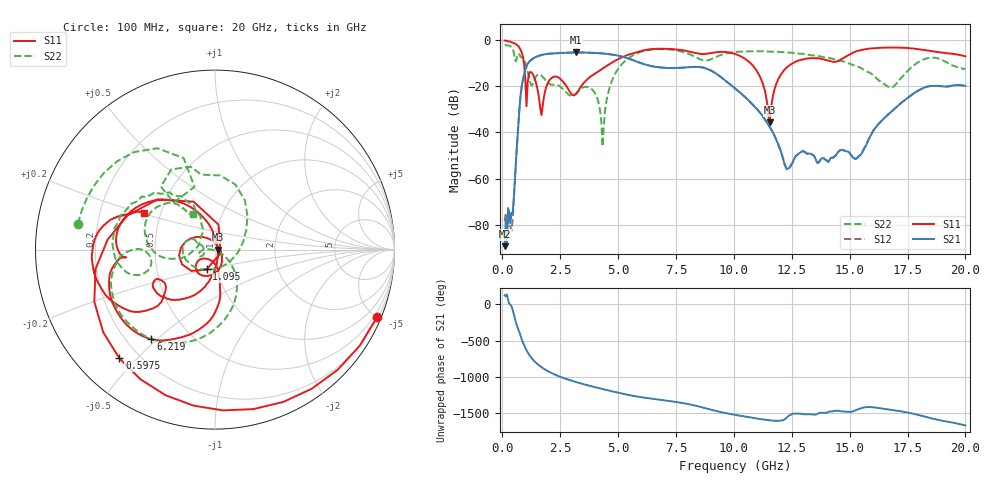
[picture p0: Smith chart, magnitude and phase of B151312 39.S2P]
!  2-Port S-parameters saved by WinCal
! VAR MeasName=S-Parameters (CALIBRATED_DATA) read from VNA (N5244A)
! VAR MeasDate=12/8/2015 5:46:42 PM
! VAR NAME=B151312 39
! VAR FILENAME=B151312 39.S2P
! VAR DATE=12/8/2015 5:46:42 PM
! VAR PHYS_PORTS=1,2
# Hz S DB R 50
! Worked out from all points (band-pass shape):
!   401 points, 100 MHz to 20 GHz, reference 50 ohm
!   highest |S21| = -5.39 dB at 3.184 GHz (marker M1); lowest = -89.2 dB at 100 MHz (marker M2)
!   |S21| within 3 dB of the highest: 1.273 GHz to 5.558 GHz (4.285 GHz wide, 125 % of centre)
!   lowest |S11| = -35.6 dB at 11.54 GHz (marker M3), VSWR 1.03, Z = 51.7 - j0.116 ohm
!   |S11| at or under -10 dB: 935.4 MHz to 4.702 GHz (3.766 GHz wide, 134 % of centre); 10.72 GHz to 12.55 GHz (1.837 GHz wide, 15.8 % of centre)
!   |S22| runs from -46.1 to -2.2 dB; largest |S21 - S12| = 0.0016
!   S11 on the Smith chart (normalised r, x): 100 MHz: 0.29, -4.99; 597.5 MHz: 0.13, -0.45; 1.095 GHz: 0.89, -0.20; 6.219 GHz: 0.30, -0.48; 20 GHz: 0.40, +0.21
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1e8  -0.20 -22.6  -89.17 129.9  -78.41 174.8  -2.19 169.3
3.985e8  -0.94 -87.1  -74.72 -23.4  -82.54 -30.4  -3.03 129.7
5.975e8  -1.86 -131.3  -51.10 100.7  -51.24 99.6  -9.16 131.2
8.4625e8  -5.63 158.5  -19.62 -128.2  -19.62 -128.2  -7.56 96.4
1.095e9  -18.46 -112.6  -10.30 59.1  -10.30 59.1  -13.68 32.5
1.493e9  -19.97 135.1  -7.13 -95.7  -7.13 -95.7  -15.24 -161.2
1.891e9  -20.54 -69.3  -6.09 172.9  -6.09 172.9  -17.66 154.2
2.43825e9  -16.30 -133.2  -5.66 89.2  -5.66 89.2  -19.79 161.9
3.1845e9  -23.28 -100.2  -5.39 8.2  -5.39 8.3  -23.23 -156.7
3.43325e9  -19.62 -82.9  -5.41 -14.7  -5.41 -14.7  -20.82 -155.2
4.32875e9  -12.36 -83.0  -5.82 -88.2  -5.81 -88.2  -46.09 -131.1
4.92575e9  -8.66 -91.5  -6.60 -133.2  -6.60 -133.2  -13.67 -54.3
6.21925e9  -4.24 -125.7  -10.74 148.6  -10.73 148.5  -4.49 -120.7
6.7665e9  -3.77 -142.2  -11.81 125.7  -11.81 125.6  -3.94 -142.2
1.005e10  -6.03 152.1  -20.91 -85.4  -20.93 -85.6  -5.20 -172.7
1.15425e10  -35.62 -3.9  -37.48 -160.1  -37.51 -160.0  -5.02 164.1
1.228875e10  -11.91 -110.9  -55.79 -120.4  -55.93 -121.5  -5.42 152.9
1.338325e10  -7.85 -144.4  -49.62 -78.2  -49.57 -77.3  -6.64 138.2
1.53235e10  -4.77 -143.3  -51.02 -12.2  -50.99 -12.7  -11.37 115.8
1.67165e10  -3.28 -172.0  -31.77 -11.7  -31.71 -12.7  -20.40 153.3
1.835825e10  -4.56 163.1  -20.12 -118.4  -20.17 -118.6  -7.87 165.7
2e10  -7.06 152.3  -19.85 128.5  -19.91 128.2  -12.72 122.1
